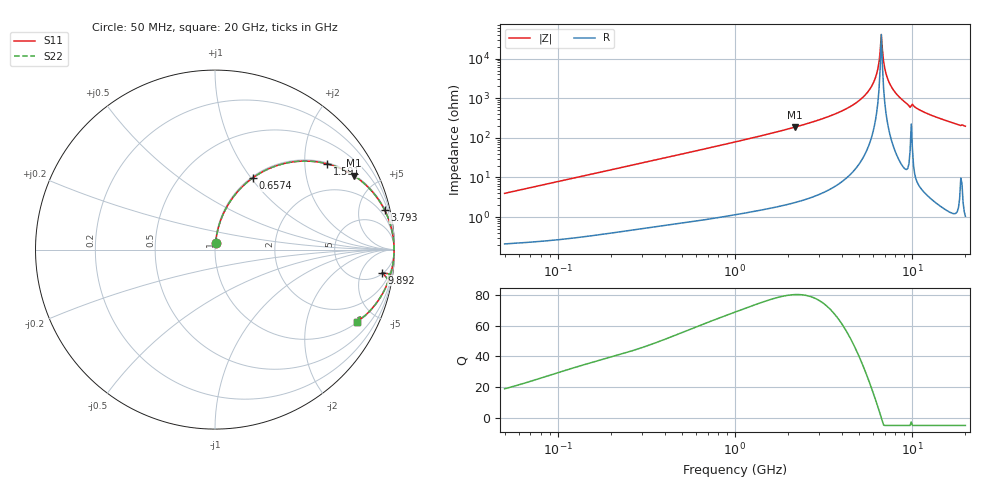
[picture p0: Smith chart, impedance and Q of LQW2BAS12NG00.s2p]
!Murata Part Number: LQW2BAS12NG00
!These Parameters are Measured in Series Mode Connection
!  o--[Z]--o
!Port1  Port2
!  o-------o
!Freq. Start=50[MHz] Stop=20[GHz], 401[Steps]
# Hz S RI R 50
!Freq.(Hz) S11(Real) S11(Imag) S21(Real) S21(Imag) S12(Real) S12(Imag) S22(Real) S22(Imag)
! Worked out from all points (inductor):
!   401 points, 50 MHz to 20 GHz, reference 50 ohm
!   read as one part in series: L = 12.6 nH near 51.52 MHz
!   highest Q = 80.3 at 2.179 GHz (marker M1), where L = 13.6 nH
!   self-resonance near 6.701 GHz
!   S11 on the Smith chart (normalised r, x): 50 MHz: 1.00, +0.08; 657.4 MHz: 1.02, +1.02; 1.591 GHz: 1.03, +2.58; 3.793 GHz: 1.13, +8.51; 9.892 GHz: 5, -12; 20 GHz: 1.02, -3.93
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5e7  0.00365 0.0394  0.9963 -0.0394  0.9963 -0.0394  0.00365 0.0394
1.364002e8  0.0143 0.1051  0.9857 -0.1051  0.9857 -0.1051  0.0143 0.1051
3.721004e8  0.0818 0.2642  0.9182 -0.2642  0.9182 -0.2642  0.0818 0.2642
6.574395e8  0.2115 0.4003  0.7885 -0.4003  0.7885 -0.4003  0.2115 0.4003
1e9  0.3836 0.4791  0.6164 -0.4791  0.6164 -0.4791  0.3836 0.4791
1.590961e9  0.6237 0.478  0.3763 -0.478  0.3763 -0.478  0.6237 0.478
2.179053e9  0.7736 0.4123  0.2264 -0.4123  0.2264 -0.4123  0.7736 0.4123
2.728004e9  0.8587 0.342  0.1413 -0.342  0.1413 -0.342  0.8587 0.342
3.792786e9  0.9446 0.2211  0.0554 -0.2211  0.0554 -0.2211  0.9446 0.2211
4.81993e9  0.9802 0.1286  0.0198 -0.1286  0.0198 -0.1286  0.9802 0.1286
5.683258e9  0.9932 0.0645  0.00683 -0.0645  0.00683 -0.0645  0.9932 0.0645
6.217679e9  0.9966 0.0295  0.00339 -0.0295  0.00339 -0.0295  0.9966 0.0295
6.406762e9  0.9972 0.0178  0.0028 -0.0178  0.0028 -0.0178  0.9972 0.0178
6.503449e9  0.9974 0.012  0.00261 -0.012  0.00261 -0.012  0.9974 0.012
6.701223e9  0.9976 0.000273  0.00244 -0.000273  0.00244 -0.000273  0.9976 0.000273
6.905011e9  0.9975 -0.0114  0.00254 0.0114  0.00254 0.0114  0.9975 -0.0114
7.114996e9  0.9971 -0.0232  0.00292 0.0232  0.00292 0.0232  0.9971 -0.0232
7.442007e9  0.996 -0.0408  0.00401 0.0408  0.00401 0.0408  0.996 -0.0408
8.389408e9  0.9898 -0.0883  0.0102 0.0883  0.0102 0.0883  0.9898 -0.0883
9.892087e9  0.9316 -0.1284  0.0684 0.1284  0.0684 0.1284  0.9316 -0.1284
1.354865e10  0.9182 -0.2706  0.0818 0.2706  0.0818 0.2706  0.9182 -0.2706
2e10  0.7933 -0.4023  0.2067 0.4023  0.2067 0.4023  0.7933 -0.4023
